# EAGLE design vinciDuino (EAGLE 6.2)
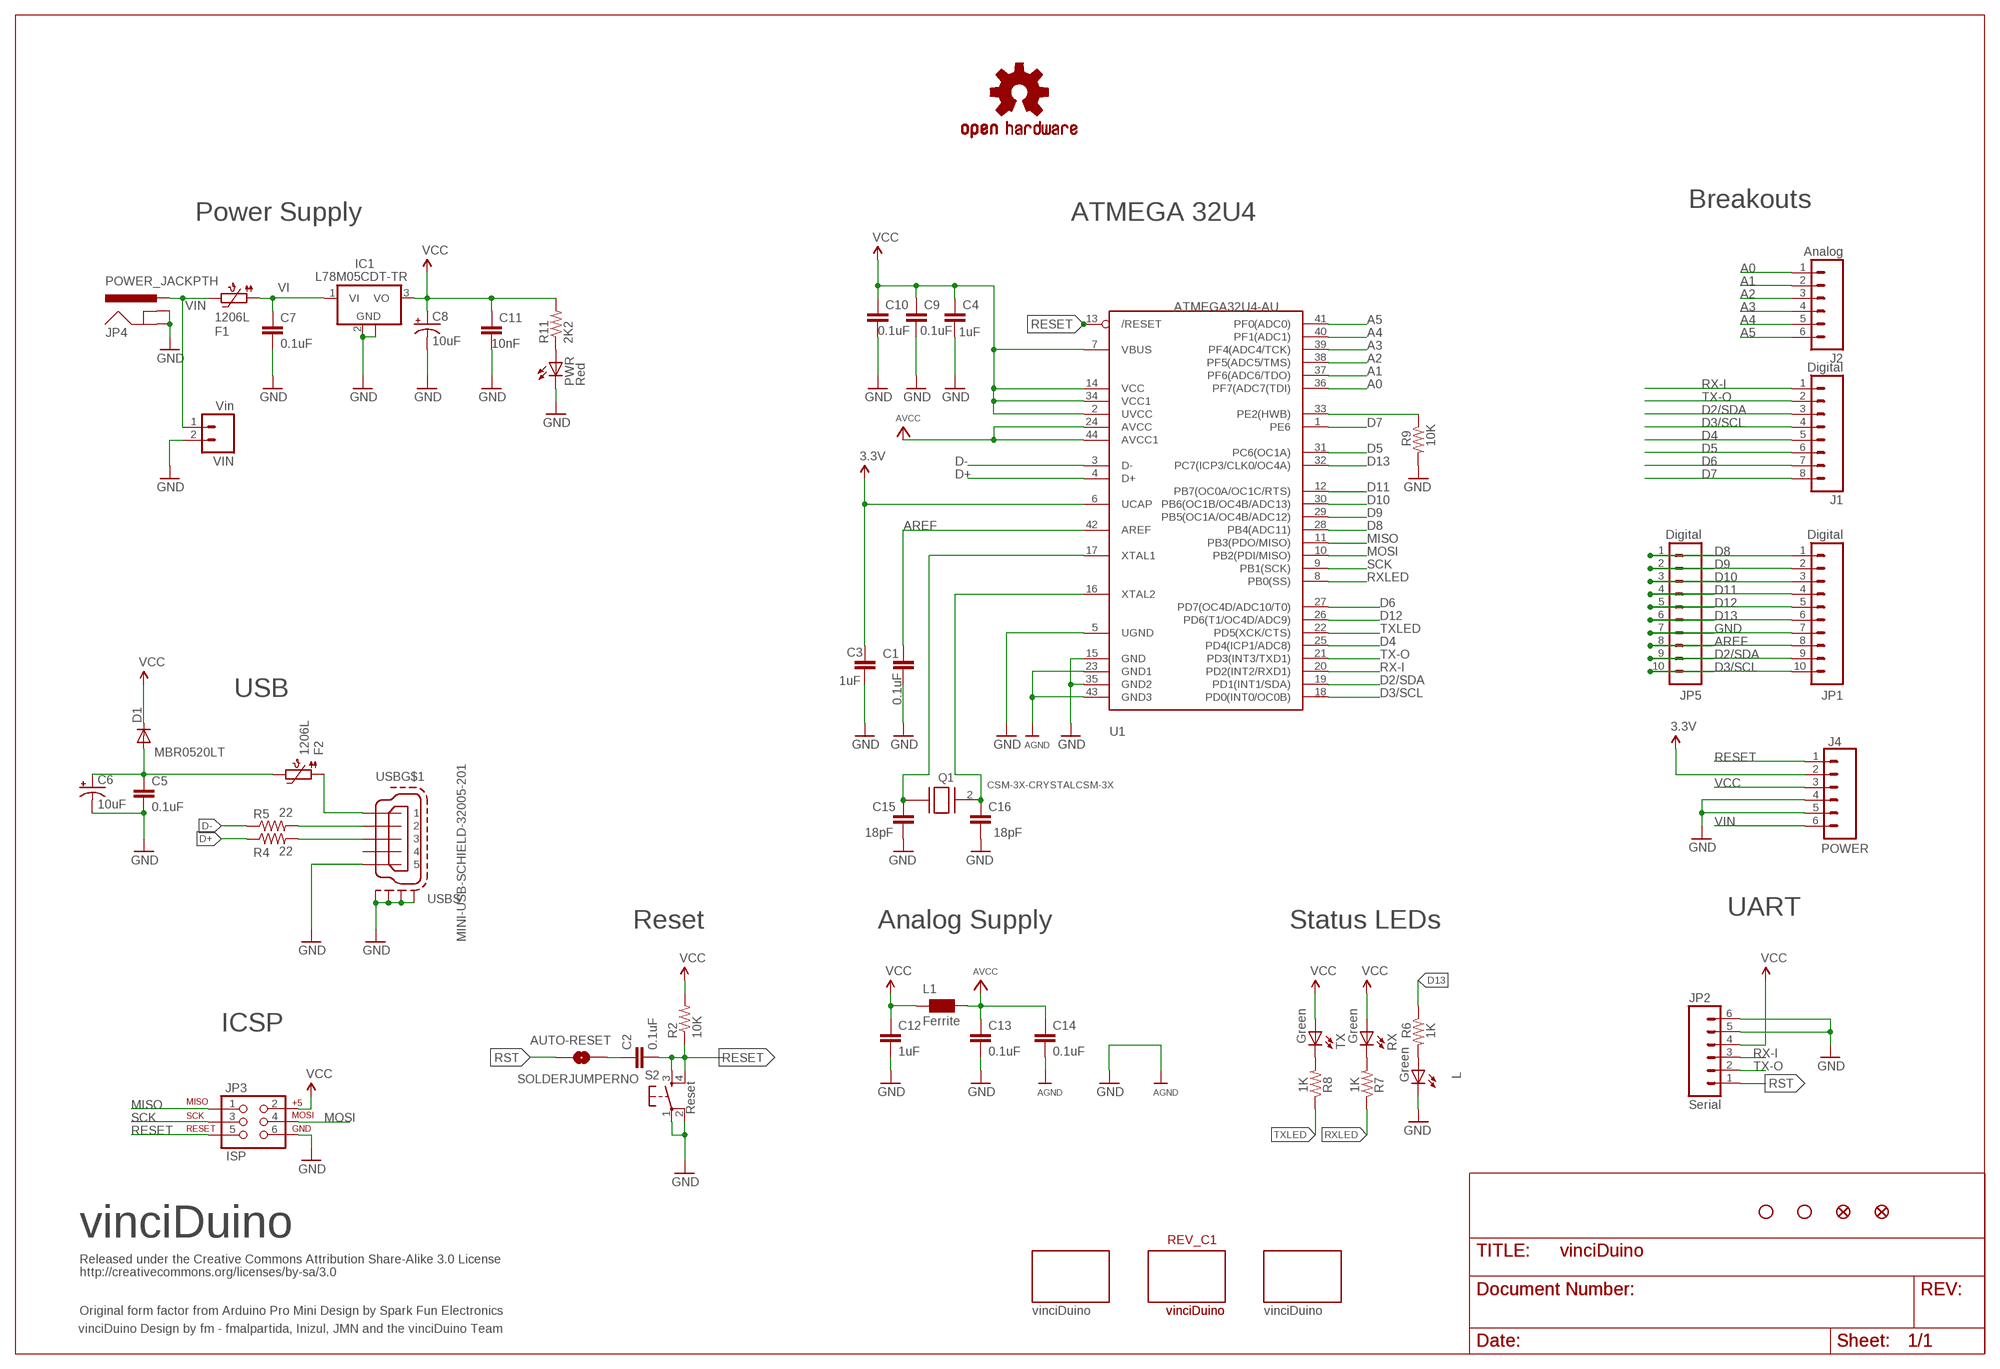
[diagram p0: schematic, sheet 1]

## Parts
AUTO-RESET  SOLDERJUMPERNO  [SJ_2S-NO]
C1  0.1uF  CAP1206  [1206]
C2  0.1uF  CAP1206  [1206]
C3  1uF  CAP1206  [1206]
C4  1uF  CAP1206  [1206]
C5  0.1uF  CAP1206  [1206]
C6  10uF  CAP_POL1206  [EIA3216]
C7  0.1uF  CAP1206  [1206]
C8  10uF  CAP_POL1206  [EIA3216]
C9  0.1uF  CAP1206  [1206]
C10  0.1uF  CAP1206  [1206]
C11  10nF  CAP1206  [1206]
C12  1uF  CAP1206  [1206]
C13  0.1uF  CAP1206  [1206]
C14  0.1uF  CAP1206  [1206]
C15  18pF  CAP1206  [1206]
C16  18pF  CAP1206  [1206]
D1  MBR0520LT  [SOD123]
F1  1206L  PTC1206_L  [1206_PTC]
F2  1206L  PTC1206_L  [1206_PTC]
IC1  L78M05CDT-TR  78XX  [SOT-223-DPAK]
J1  Digital  M081X08  [1X08]
J2  Analog  M06SIP  [1X06]
J4  POWER  M06SIP  [1X06]
JP1  Digital  M10"  [1X10]
JP2  Serial  M06SIP  [1X06]
JP3  ISP  AVR_SPI_PRG_6PTH  [2X3]
JP4  POWER_JACKPTH  [POWER_JACK_PTH]
JP5  Digital  M10"  [1X10]
L  Green  LED1206  [LED-1206]
L1  Ferrite  WE-CBF_1206W  [1206W]
PWR  Red  LED1206  [LED-1206]
Q1  CSM-3X-CRYSTALCSM-3X  [CSM-3X]
R2  10K  R-US_R1206  [R1206]
R4  22  R-US_R1206  [R1206]
R5  22  R-US_R1206  [R1206]
R6  1K  R-US_R1206  [R1206]
R7  1K  R-US_R1206  [R1206]
R8  1K  R-US_R1206  [R1206]
R9  10K  R-US_R1206  [R1206]
R11  2K2  R-US_R1206  [R1206]
REV_C1  vinciDuino  BOARD_INFO_  [ARDUINO_FORUM]
RX  Green  LED1206  [LED-1206]
S2  Reset  TAC_SWITCHSMD  [TACTILE_SWITCH_SMD]
TX  Green  LED1206  [LED-1206]
U1  ATMEGA32U4-AU  [TQFP44]
U$1  VINCIDUINO_  VINCIDUINO_25  [VINCIDUINO]
U$2  FIDUCIAL1X2  [FIDUCIAL-1X2]
U$3  VINCIDUINO_15  [VINCIDUINO_VSMAL]
U$4  FIDUCIAL1X2  [FIDUCIAL-1X2]
U$9  STAND-OFF  [STAND-OFF]
U$10  STAND-OFF  [STAND-OFF]
U$14  OSHW-LOGOS  [OSHW-LOGO-S]
USB  MINI-USB-SCHIELD-32005-201  [32005-201]
VIN  Vin  M021X02_NO_SILK  [1X02_NO_SILK]

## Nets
3.3V: C3.1 J4.2 U1.6(UCAP)
A0: J2.1 U1.36(PF7(ADC7(TDI))
A1: J2.2 U1.37(PF6(ADC6/TDO))
A2: J2.3 U1.38(PF5(ADC5/TMS))
A3: J2.4 U1.39(PF4(ADC4/TCK))
A4: J2.5 U1.40(PF1(ADC1))
A5: J2.6 U1.41(PF0(ADC0))
AREF: C1.2 JP1.8 JP5.8 U1.42(AREF)
AVCC: C13.1 C14.1 L1.2 U1.24(AVCC) U1.44(AVCC1)
D2/SDA: J1.3 JP1.9 JP5.9 U1.19(PD1(INT1/SDA))
D3/SCL: J1.4 JP1.10 JP5.10 U1.18(PD0(INT0/OC0B))
D4: J1.5 U1.25(PD4(ICP1/ADC8))
D5: J1.6 U1.31(PC6(OC1A))
D6: J1.7 U1.27(PD7(OC4D/ADC10/T0))
D7: J1.8 U1.1(PE6)
D8: JP1.1 JP5.1 U1.28(PB4(ADC11))
D9: JP1.2 JP5.2 U1.29(PB5(OC1A/OC4B/ADC12))
D10: JP1.3 JP5.3 U1.30(PB6(OC1B/OC4B/ADC13))
D11: JP1.4 JP5.4 U1.12(PB7(OC0A/OC1C/RTS))
D12: JP1.5 JP5.5 U1.26(PD6(T1/OC4D/ADC9))
D13: JP1.6 JP5.6 R6.1 U1.32(PC7(ICP3/CLK0/OC4A))
D+: R4.1 U1.4(D+)
D-: R5.1 U1.3(D-)
GND: C1.1 C3.2 C4.2 C5.2 C6.C(-) C7.2 C8.C(-) C9.2 C10.2 C11.2 C12.2 C13.2 C14.2 C15.2 C16.2 IC1.2(GND) IC1.4(GND) J4.4 J4.5 JP1.7 JP2.5 JP2.6 JP3.6 JP4.GND JP4.GNDBREAK JP5.7 L.C PWR.C R9.2 S2.1 S2.2 U1.5(UGND) U1.15(GND) U1.23(GND1) U1.35(GND2) U1.43(GND3) USB.5 USB.M1(S:S1) USB.M2(S:S2) USB.M3(S:S3) USB.M4(S:S4) VIN.2 ; supply symbol labelled AGND
MISO: JP3.1 U1.11(PB3(PDO/MISO))
MOSI: JP3.4 U1.10(PB2(PDI/MISO))
N$1: R8.2 TX.C
N$2: R5.2 USB.2
N$3: C16.1 Q1.2 U1.16(XTAL2)
N$4: C15.1 Q1.1 U1.17(XTAL1)
N$5: R4.2 USB.3
N$6: R9.1 U1.33(PE2(HWB))
N$7: L.A R6.2
N$8: AUTO-RESET.2 C2.1
N$9: R7.2 RX.C
N$13: F2.1 USB.1
N$38: PWR.A R11.1
RESET: C2.2 J4.1 JP3.5 R2.1 S2.3 S2.4 U1.13(/RESET)
RST: AUTO-RESET.1 JP2.1
RX-I: J1.1 JP2.3 U1.20(PD2(INT2/RXD1))
RXLED: R7.1 U1.8(PB0(SS))
SCK: JP3.3 U1.9(PB1(SCK))
TX-O: J1.2 JP2.2 U1.21(PD3(INT3/TXD1))
TXLED: R8.1 U1.22(PD5(XCK/CTS))
VBUS: C5.1 C6.A(+) D1.A F2.2
VCC: C4.1 C8.A(+) C9.1 C10.1 C11.1 C12.1 D1.C IC1.3(VO) J4.3 JP2.4 JP3.2 L1.1 R2.2 R11.2 RX.A TX.A U1.2(UVCC) U1.7(VBUS) U1.14(VCC) U1.34(VCC1)
VI [vcc]: C7.1 F1.1 IC1.1(VI)
VIN [vcc]: F1.2 J4.6 JP4.PWR VIN.1
Unconnected: USB.4

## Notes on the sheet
- Breakouts
- Power Supply | ATMEGA 32U4
- USB
- UART
- Reset | Analog Supply | Status LEDs
- ICSP
- vinciDuino
- Released under the Creative Commons Attribution Share-Alike 3.0 License
- http://creativecommons.org/licenses/by-sa/3.0
- Original form factor from Arduino Pro Mini Design by Spark Fun Electronics
- vinciDuino Design by fm - fmalpartida, Inizul, JMN and the vinciDuino Team

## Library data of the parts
AUTO-RESET = SparkFun:SOLDERJUMPER: Solder Jumper
C1-C5 C7 C9-C16 = sparkfun_2:CAP: Capacitor
C6 C8 = SparkFun:CAP_POL: Capacitor Polarized
D1 = diode:MBR0520LT: SCHOTTKY BARRIER RECTIFIER
F1 F2 = microbuilder:PTC: PTC (Resettable Fuse)
IC1 = fmc:78XX
J1 = SparkFun:M08: Header 8 Standard 8-pin 0.1" header. Use with straight break away headers (SKU : PRT-00116), right angle break away headers (PRT-00553), swiss pins (PRT-00743), machine pins (PRT-00117), and female headers (PRT-00115).
J2 J4 JP2 = SparkFun:M06: Header 6 Standard 6-pin 0.1" header. Use with straight break away headers (SKU : PRT-00116), right angle break away headers (PRT-00553), swiss pins (PRT-00743), machine pins (PRT-00117), and female headers (PRT-00115). Molex polarized connector foot print use with SKU : PRT-08094 with associated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
JP1 JP5 = SparkFun:M10: Header 10 Standard 10-pin 0.1" header. Use with straight break away headers (SKU : PRT-00116), right angle break away headers (PRT-00553), swiss pins (PRT-00743), machine pins (PRT-00117), and female headers (PRT-00115).
JP3 = SparkFun:AVR_SPI_PRG_6: AVR ISP 6 Pin This is the reduced ISP connector for AVR programming. Common on Arduino. This footprint will take up less PCB space and can be used with a 10-pin to 6-pin adapter such as SKU: BOB-08508
JP4 = SparkFun:POWER_JACK: Power Jack This is the standard 5.5mm barrel jack for power. The PTH is the most common, proven, reliable, footprint. All others are experimental. The Slot footprint only works if the mill layer is transmitted to the PCB fab house so be warned. Spark Fun Electronics SKU : PRT-00119. Mating wall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
L PWR RX TX = SparkFun:LED: LEDs
L1 = wuerth-elektronik:WE-CBF: SMD EMI Suppression Ferrite Beads
Q1 = fmc:CSM-3X-CRYSTAL
R2 R4-R9 R11 = adafruit:R-US_: RESISTOR, American symbol
REV_C1 = fmc:BOARD_INFO_
S2 = SparkFun:TAC_SWITCH: Momentary Switch Button commonly used for reset or general input. Spark Fun Electronics SKU : COM-00097
U1 = adafruit:ATMEGA32U4: http://www.ladyada.net/library/eagle
U$1 U$3 = fmc:VINCIDUINO_
U$2 U$4 = SparkFun:FIDUCIAL: Fiducial Alignment Points
U$9 U$10 = SparkFun:STAND-OFF: Stand Off
U$14 = SparkFun:OSHW-LOGO: Open Source Hardware Logo This logo indicates the piece of hardware it is found on incorporates a OSHW license and/or adheres to the definition of open source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
USB = con-cypressindustries:MINI-USB-SCHIELD-: MINI USB-B Conector Source: www.cypressindustries.com; OC_FARNELL: unknown; OC_NEWARK: unknown
VIN = SparkFun:M02: Header 2

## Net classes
1 vcc: width 0.254 mm

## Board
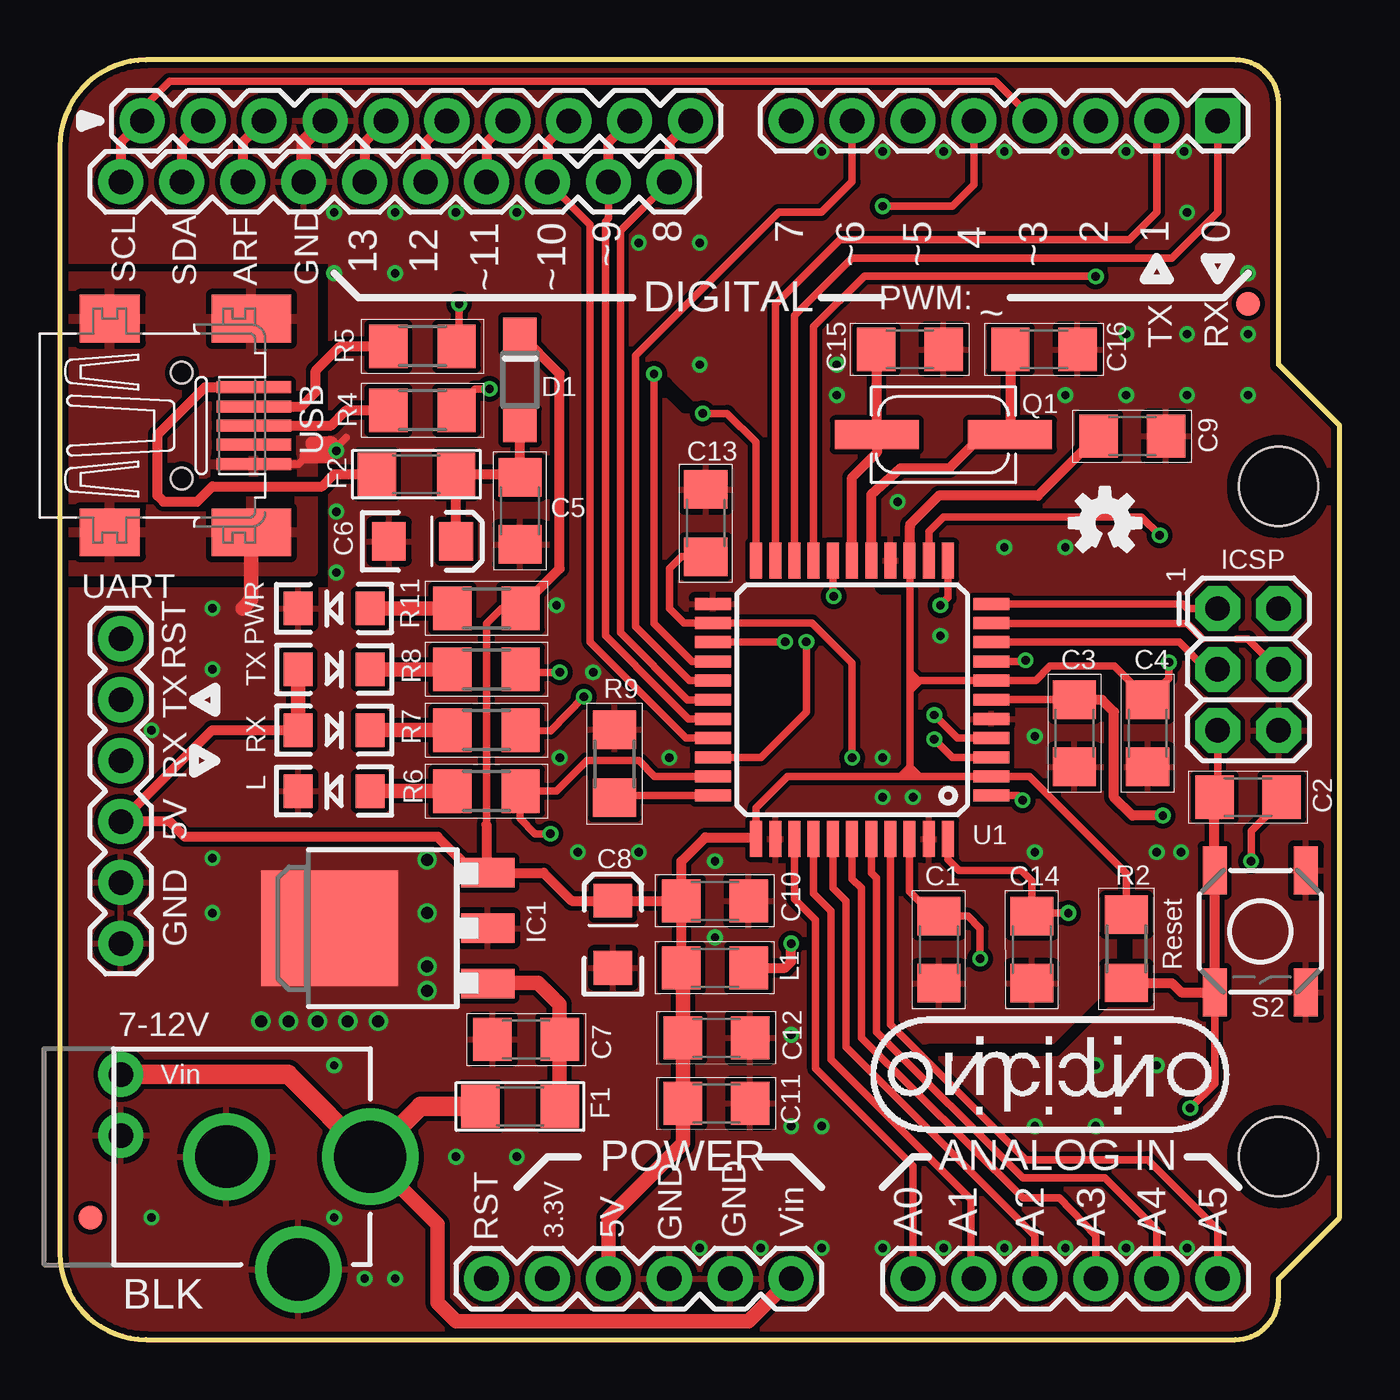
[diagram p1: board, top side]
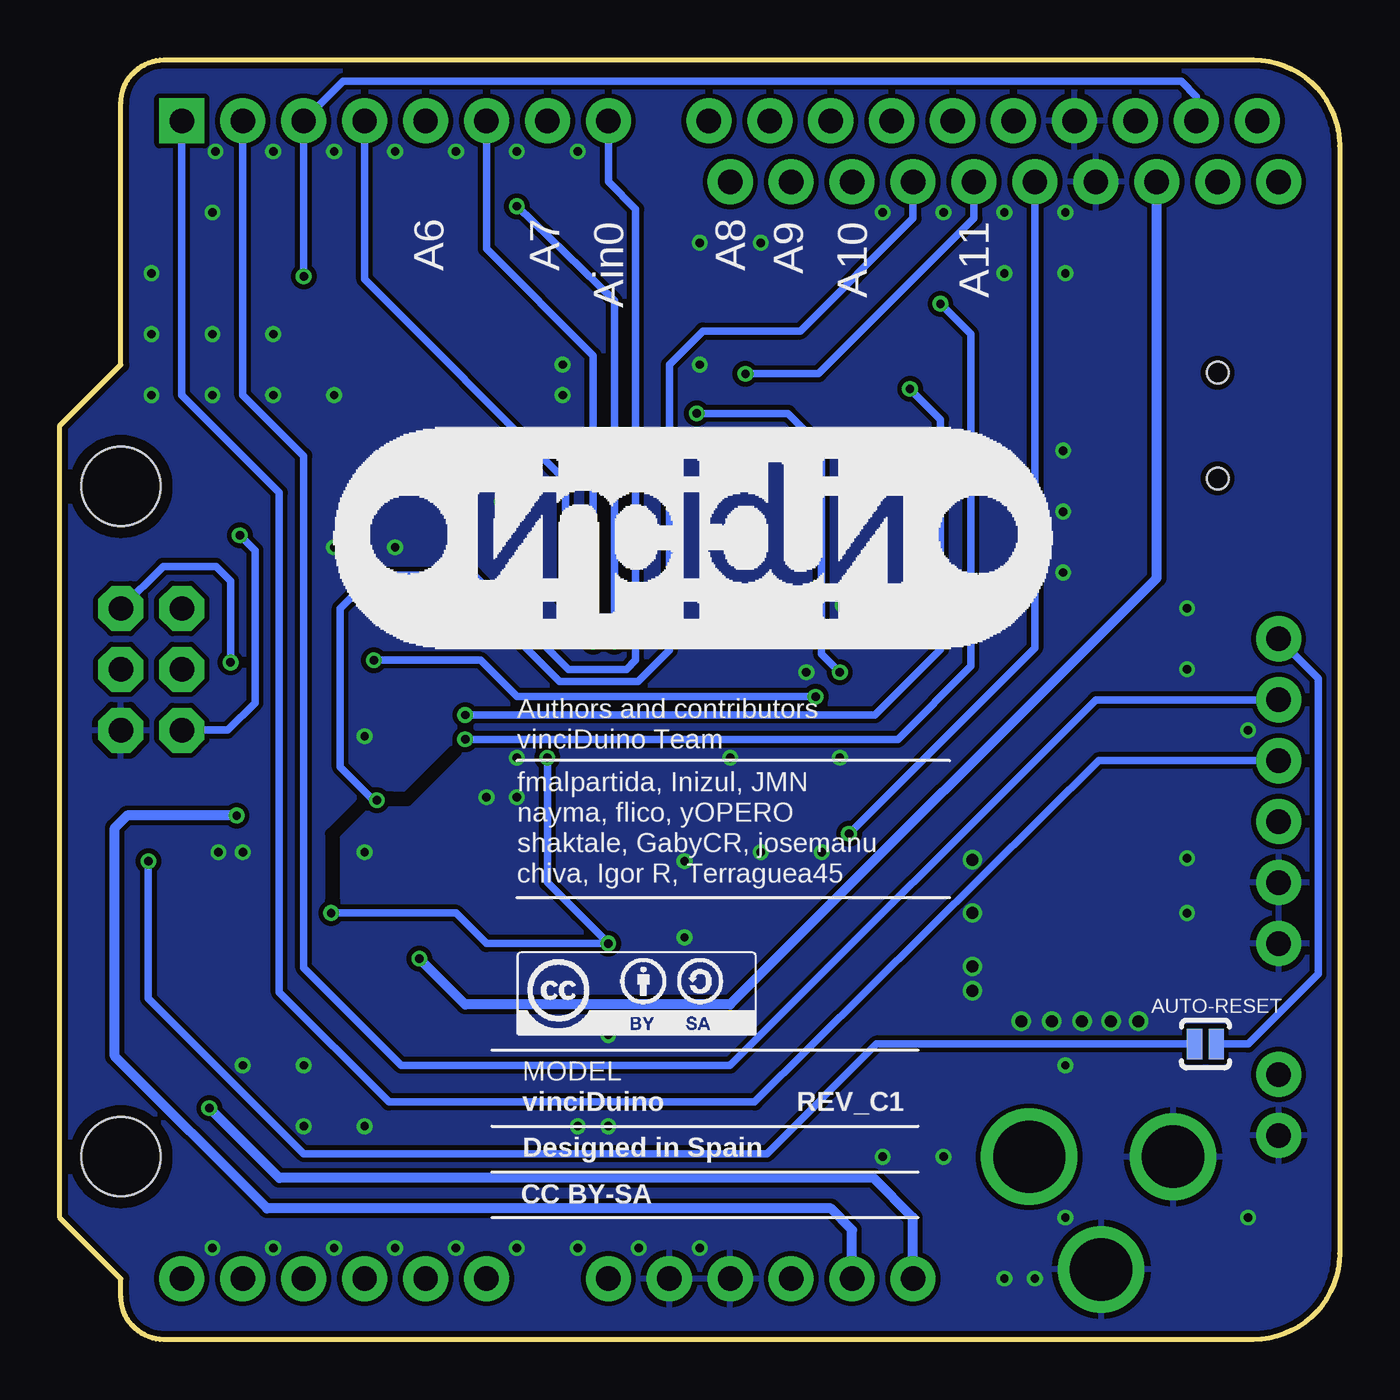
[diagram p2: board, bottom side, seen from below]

Size 53.34 x 53.34 mm. Coordinates in mm from the lower left corner, seen from the top.
Outline: 50.8,40.64 50.8,51.54 arc90 49,53.34 3.59,53.34 arc90 0,49.75 0,3.59 arc90 3.59,0 49,0 arc90 50.8,1.8 50.8,2.54 53.34,5.08 53.34,38.1 50.8,40.64
Copper layers (1*16): Top 0.0356mm / dielectric 1.5011mm / Bottom 0.0356mm
Design rules: minimum track width 6mil, minimum drill 0.35mm, track to track 8mil, track to pad 8mil, pad to pad 8mil, via to via 8mil, smd to smd 8mil, copper to edge 10mil, drill to drill 6mil, minimum pad ring 12mil, minimum via ring 6mil, stop-mask expansion 4mil, vias tented up to drill 25mil, thermal gap 10mil
tRestrict: area 34.3,31.4 to 34.9,31.5; area 25.1,38.9 to 26.2,39.9; area 36.2,12.1 to 43.4,14; area 44.3,15.9 to 44.5,16.8
bRestrict: area 36.8,22.5 to 39.5,24.5; area 40.6,18.3 to 42,22.4

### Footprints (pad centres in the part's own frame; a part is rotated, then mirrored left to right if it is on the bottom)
SJ_2S-NO = smd 0.635 x 1.27: 1 -0.45,0; 2 0.45,0
1206 = smd 1.6 x 1.8: 1 -1.4,0; 2 1.4,0
EIA3216 = smd 1.4 x 1.6: A 1.4,0; C -1.4,0
SOD123 = smd 1.4 x 1.4: A 1.9,0; C -1.9,0
1206_PTC = smd 1.6 x 1.8: 1 -1.654,0; 2 1.654,0
SOT-223-DPAK = smd 1.219 x 2.235: 1 -2.311,-3.099; 2 0,-3.099; 3 2.311,-3.099 | smd 4.826 x 5.715: 4 0,3.493
1X08@1 = drill 1.016 pad 1.88 square: 1 0,0 | drill 1.016 pad 1.88: 2 2.54,0; 3 5.08,0; 4 7.62,0; 5 10.16,0; 6 12.7,0; 7 15.24,0; 8 17.78,0
1X06@1 = drill 1.016 pad 1.88: 1 -6.35,0; 2 -3.81,0; 3 -1.27,0; 4 1.27,0; 5 3.81,0; 6 6.35,0
1X10 = drill 1.016 pad 1.88: 1 0,0; 2 2.54,0; 3 5.08,0; 4 7.62,0; 5 10.16,0; 6 12.7,0; 7 15.24,0; 8 17.78,0; 9 20.32,0; 10 22.86,0
2X3@1 = drill 1.016 pad 1.88 octagon: 1 0,0; 2 0,2.54; 3 2.54,0; 4 2.54,2.54; 5 5.08,0; 6 5.08,2.54
POWER_JACK_PTH@1 = drill 2.6: GND 0,7.7; GNDBREAK 4.7,10.7 | drill 3: PWR 0,13.7
LED-1206 = smd 1.2 x 1.4: A -1.5,0; C 1.5,0
1206W = smd 1.6 x 1.8: 1 -1.4,0; 2 1.4,0
CSM-3X = smd 3.5 x 1.2: 1 2.775,0; 2 -2.775,0
R1206 = smd 1.6 x 1.803: 1 -1.422,0; 2 1.422,0
TACTILE_SWITCH_SMD@1 = smd 2 x 1: 1 -2.54,1.905; 2 2.54,1.905; 3 -2.54,-1.905; 4 2.54,-1.905
TQFP44 = smd 1.5 x 0.5: 1 -5.8,4; 2 -5.8,3.2; 3 -5.8,2.4; 4 -5.8,1.6; 5 -5.8,0.8; 6 -5.8,0; 7 -5.8,-0.8; 8 -5.8,-1.6; 9 -5.8,-2.4; 10 -5.8,-3.2; 11 -5.8,-4; 23 5.8,-4; 24 5.8,-3.2; 25 5.8,-2.4; 26 5.8,-1.6; 27 5.8,-0.8; 28 5.8,0; 29 5.8,0.8; 30 5.8,1.6; 31 5.8,2.4; 32 5.8,3.2; 33 5.8,4 | smd 0.5 x 1.5: 12 -4,-5.8; 13 -3.2,-5.8; 14 -2.4,-5.8; 15 -1.6,-5.8; 16 -0.8,-5.8; 17 0,-5.8; 18 0.8,-5.8; 19 1.6,-5.8; 20 2.4,-5.8; 21 3.2,-5.8; 22 4,-5.8; 34 4,5.8; 35 3.2,5.8; 36 2.4,5.8; 37 1.6,5.8; 38 0.8,5.8; 39 0,5.8; 40 -0.8,5.8; 41 -1.6,5.8; 42 -2.4,5.8; 43 -3.2,5.8; 44 -4,5.8
FIDUCIAL-1X2 = smd 1 x 1: 1 0,0
STAND-OFF@1 = hole 3.302: 0,0
32005-201 = smd 3.1 x 0.5: 1 3,1.6; 2 3,0.8; 3 3,0; 4 3,-0.8; 5 3,-1.6 | smd 2.5 x 2: M1 -3,-4.45; M2 -3,4.45 | smd 3.3 x 2: M3 2.9,4.45; M4 2.9,-4.45 | hole 0.9: 0,2.2; 0,-2.2
1X02_NO_SILK = drill 1.016 pad 1.88: 1 0,0; 2 2.54,0

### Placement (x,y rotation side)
AUTO-RESET  5.59,12.32 180 bottom
C1  36.64,16.26 90 top
C2  49.53,22.61 180 top
C3  42.29,25.27 270 top
C4  45.34,25.27 270 top
C5  19.18,34.54 270 top
C6  15.11,33.27 0 top
C7  19.43,12.51 180 top
C8  23.05,16.89 90 top
C9  44.7,37.66 0 top
C10  27.3,18.29 0 top
C11  27.37,9.84 0 top
C12  27.37,12.57 0 top
C13  26.92,34.04 90 top
C14  40.51,16.26 270 top
C15  35.43,41.27 0 top
C16  41.02,41.27 0 top
D1  19.18,40.01 270 top
F1  19.18,9.72 180 top
F2  14.86,36.07 0 top
IC1  14.73,17.14 90 top
J1  Digital  [1X08@1]  48.26,50.8 180 top
J2  Analog  [1X06@1]  41.91,2.54 0 top
J4  POWER  [1X06@1]  24.13,2.54 0 top
JP1  26.29,50.8 180 top
JP2  Serial  [1X06@1]  2.54,22.86 270 top
JP3  ISP  [2X3@1]  48.26,30.47 270 top
JP4  POWER_JACKPTH  [POWER_JACK_PTH@1]  -0.76,7.62 270 top
JP5  25.4,48.26 180 top
L  11.43,22.86 180 top
L1  27.3,15.49 0 top
PWR  11.43,30.48 180 top
Q1  36.83,37.72 180 top
R2  44.45,16.29 90 top
R4  15.11,38.73 180 top
R5  15.11,41.4 180 top
R6  17.78,22.86 180 top
R7  17.78,25.4 180 top
R8  17.78,27.94 180 top
R9  23.11,24 90 top
R11  17.78,30.48 0 top
REV_C1  26.67,8.89 0 bottom
RX  11.43,25.4 0 top
S2  Reset  [TACTILE_SWITCH_SMD@1]  50.04,17.02 270 top
TX  11.43,27.94 0 top
U1  33.02,26.67 180 top
U$1  41.91,28.83 0 bottom
U$2  1.27,5.08 0 top
U$3  33.78,8.64 0 top
U$4  49.53,43.18 0 top
U$9  STAND-OFF  [STAND-OFF@1]  50.8,35.56 0 top
U$10  STAND-OFF  [STAND-OFF@1]  50.8,7.62 0 top
U$13  [SA-BY]  34.29,12.7 0 bottom
U$14  43.56,34.04 0 top
USB  5.08,38.1 0 top
VIN  2.54,11.05 270 top

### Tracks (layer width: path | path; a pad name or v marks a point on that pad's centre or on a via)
3.3V  (via drill 0.35)
  Top 0.305: C3.1 U1.6
  Top 0.406: v45.97,21.84 44.7,21.84 43.94,22.61 43.94,26.16 43.43,26.67 C3.1
  Bottom 0.406: J4.2 20.32,4.57 21.21,5.46 44.7,5.46 51.05,11.81 51.05,21.34 50.55,21.84 v45.97,21.84
A0
  Top 0.305: U1.36 30.62,18.37 31.5,17.49 31.5,11.3 35.56,7.24 J2.1
A1
  Top 0.305: U1.37 31.42,18.59 32.13,17.88 32.13,11.68 37.97,5.84 37.97,2.67 J2.2
A2
  Top 0.305: U1.38 32.22,18.83 32.77,18.29 32.77,12.19 40.64,4.32 J2.3
A3
  Top 0.305: U1.39 33.02,19.21 33.4,18.83 33.4,12.57 40.13,5.91 41.66,5.91 43.18,4.32 J2.4
A4
  Top 0.305: 33.78,20.83 U1.40 33.82,19.46 34.04,19.24 34.04,12.83 40.13,6.73 43.56,6.73 45.72,4.57 J2.5
A5
  Top 0.305: U1.41 34.62,13.13 40.26,7.49 45.34,7.49 48.26,4.57 J2.6
AREF  (via drill 0.35)
  Top 0.305: U1.42 35.42,18.68 36.58,17.53 36.64,17.53 C1.2 37.85,17.65 38.35,17.14 v38.35,15.88
  Top 0.406: JP1.8 7.62,49.91 JP5.8
  Bottom 0.406: v38.35,15.88 36.45,13.97 25.4,13.97 7.62,31.75 JP5.8
AVCC  (via drill 0.35)
  Top 0.305: U1.44 37.02,20 37.47,19.56 40.07,19.56 40.51,19.11 C14.1 40.51,17.78 v42.04,17.78 | C13.1 25.91,32.64 25.4,32.13 25.4,30.48 26.01,29.87 U1.24 31.34,29.87 33.02,28.19 v33.02,24.26
  Top 0.406: v30.48,16.51 30.48,15.75 30.23,15.49 L1.2
  Bottom 0.305: v30.48,16.51 33.02,19.05 v33.02,24.26 | v30.48,16.51 31.75,17.78 | v42.04,17.78 36.83,17.78 35.56,16.51 v30.48,16.51
D2/SDA  (via drill 0.35)
  Top 0.305: U1.19 31.42,42.22 33.53,44.32 v43.18,44.32
  Top 0.406: JP1.9 5.08,49.91 JP5.9
  Bottom 0.305: JP1.9 5.97,51.82 6.6,52.45 41.53,52.45 J1.3 v43.18,44.32
D3/SCL  (via drill 0.35)
  Top 0.305: JP1.10 3.43,51.31 4.57,52.45 38.99,52.45 J1.4 | U1.18 32.22,31.03 v32.26,30.99
  Top 0.406: JP1.10 2.54,49.91 JP5.10
  Bottom 0.305: v32.26,30.99 32.26,35.81 40.64,44.2 J1.4
D4  (via drill 0.35)
  Top 0.305: U1.25 29.6,29.07 v30.23,29.08 | v34.29,47.24 37.21,47.24 38.1,48.13 J1.5
  Bottom 0.305: v30.23,29.08 30.23,43.31 v34.29,47.24
D5  (via drill 0.35)
  Top 0.305: U1.31 29.22,24.27 31.11,26.16 v31.11,29.08
  Bottom 0.305: v31.11,29.08 31.11,41.02 35.56,45.47 J1.6
D6
  Top 0.305: 26.5,27.47 U1.27 26.25,27.47 24,29.72 24,41.02 29.97,46.99 31.75,46.99 33.02,48.26 J1.7
D7  (via drill 0.35)
  Top 0.305: U1.1 39.94,22.67 v40.13,22.48
  Bottom 0.305: v40.13,22.48 40.26,22.48 41.66,23.88 41.66,30.48 40.26,31.88 36.07,31.88 32.13,27.94 29.72,27.94 29.34,28.32 29.34,47.12 30.48,48.26 J1.8
D8
  Top 0.305: U1.28 26.16,26.67 23.37,29.46 23.37,46.23 JP5.1
  Top 0.406: JP1.1 25.4,49.91 JP5.1
D9
  Top 0.305: 25.27,26.8 22.73,29.34 22.73,46.61 22.86,46.74 JP5.2 | 25.27,26.8 | 25.27,26.8 26.19,25.88 U1.29
  Top 0.406: JP5.2 22.86,49.91 JP1.2
D10
  Top 0.305: U1.30 27.21,25.08 26.1,25.08 22.1,29.08 22.1,46.48 JP5.3
  Top 0.406: JP1.3 20.32,49.91 JP5.3
D11  (via drill 0.35)
  Top 0.305: U1.12 37.02,30.92 v36.7,30.61
  Top 0.406: JP1.4 17.78,49.91 JP5.4
  Bottom 0.305: v36.7,30.61 35.69,30.61 32.51,27.43 29.24,27.43 27.94,28.73 27.94,40.64 26.54,42.04 22.48,42.04 17.78,46.74 JP5.4
D12  (via drill 0.35)
  Top 0.305: U1.26 26.34,28.27 24.77,29.84 v24.77,40.26
  Top 0.406: JP1.5 15.24,49.91 JP5.5
  Bottom 0.305: v24.77,40.26 21.72,40.26 15.24,46.74 JP5.5
D13  (via drill 0.35)
  Top 0.305: U1.32 24.79,23.47 24.13,24.13 21.97,24.13 20.7,22.86 R6.1 19.18,22.84 19.18,21.72 19.81,21.08 v20.45,21.08
  Top 0.406: JP1.6 12.7,49.91 JP5.6
  Bottom 0.305: v20.45,21.08 12.7,28.83 JP5.6
D+  (via drill 0.35)
  Top 0.305: U1.4 37.41,25.07 v36.45,26.04 | 16.51,38.71 R4.1 17.3,39.62 v17.91,39.62
  Bottom 0.305: v36.45,26.04 19.37,26.04 16.64,28.77 16.64,38.35 v17.91,39.62
D-  (via drill 0.35)
  Top 0.305: U1.3 37.2,24.27 v36.45,25.02 | v16.64,43.18 16.64,41.5 R5.1
  Bottom 0.305: v36.45,25.02 18.41,25.02 15.37,28.07 15.37,41.91 v16.64,43.18
GND  (via drill 0.35, 0.5)
  Top 0.305: USB.5 9.96,36.5 10.29,36.83 | 11.18,36.83 11.94,37.59
  Top 0.61: 10.92,50.67 10.16,49.91 JP5.7 | 10.29,36.83 11.18,36.83 | USB.M4 7.98,30.84 7.62,30.48 | 10.54,37.34 11.3,37.34
  other vias: 22.23,27.81 24.13,20.32 21.59,20.32 24.13,45.72 39.37,49.53 26.67,45.72 11.43,44.45 11.43,46.99 40.64,8.89 43.18,8.89 46.99,39.37 49.53,39.37 34.29,49.53 46.99,46.99 30.48,12.7 39.37,33.02 41.91,33.02 41.91,49.53 49.53,44.45 13.97,46.99 13.97,44.45 11.53,31.97 26.67,3.81 29.21,3.81 3.81,5.08 46.99,41.91 49.53,41.91 6.35,20.07 6.35,17.78 26.67,40.64 10.73,13.27 12,13.27 13.27,13.27 15.3,14.54 15.3,15.56 15.3,17.78 8.38,13.27 9.53,13.27 15.3,20 45.72,20.32 46.74,20.32 40.64,25.15 16.51,7.62 19.05,7.62 11.43,11.43 34.29,24.26 36.7,29.34 43.18,11.43 45.72,11.43 34.29,22.61 35.56,22.61 36.83,3.81 39.37,3.81 41.91,3.81 44.45,3.81 46.99,3.81 27.3,19.94 27.3,16.76 31.75,8.89 30.48,8.89 40.64,20.32 11.43,5.08 12.7,2.54 13.97,2.54 20.7,30.61 6.35,30.48 6.35,27.94 11.53,34.51 44.45,49.53 36.83,49.53 46.86,49.53 31.75,49.53 16.51,46.99 19.05,46.99 31.75,3.81 34.29,3.81 25.4,24.26 20.83,24.26 3.81,25.4 44.45,41.91 44.45,39.37 32.38,39.37 34.92,34.92 32.38,40.64 41.91,39.37 11.53,37.05
  pour Top (isolate 0.203): 0,53.34 53.34,53.34 53.34,0 0,0 0,31.24 11.3,31.24 11.3,44.96 0,44.96
  pour Bottom (isolate 0.203): 0,53.34 53.34,53.34 53.34,0 15.88,0.13 10.79,0.13 0,0
  pour Top (no thermals): 7.62,20.32 15.24,20.32 15.24,13.97 7.62,13.97
  pour Top: 0,44.32 10.54,44.32 10.54,32 0,32
MISO
  Top 0.305: U1.11 46.8,30.67 46.99,30.48 JP3.1
MOSI
  Top 0.203: 47.62,29.21 49.05,29.21
  Top 0.305: U1.10 38.84,29.84 46.99,29.84 47.5,29.34 47.62,29.21 | 49.05,29.21 49.52,29.21 JP3.4
N$1
  Top 0.61: TX.C R8.2
N$2
  Top 0.305: 13.97,41.91 13.72,41.66 13.72,41.4 R5.2
  Top 0.406: USB.2 10.07,38.9 10.67,39.5 10.67,40.39 11.68,41.4 R5.2
N$3
  Top 0.406: C16.1 39.62,37.73 Q1.2 38.48,37.72 37.08,36.32 35.05,36.32 33.82,35.22 U1.16
N$4
  Top 0.406: C15.1 34.03,37.72 34.04,37.72 Q1.1 34.05,36.98 33.02,35.94 U1.17
N$5
  Top 0.406: USB.3 11.3,38.1 11.94,38.73 R4.2
N$6
  Top 0.305: U1.33 23.2,22.67 R9.1
N$7
  Top 0.61: L.A R6.2
N$8  (via drill 0.35)
  Top 0.305: C2.1 50.93,22.48 49.66,21.21 v49.66,19.94
  Bottom 0.305: AUTO-RESET.2 19.3,12.32 23.88,7.75 43.18,7.75 49.66,14.22 v49.66,19.94
N$9
  Top 0.61: RX.C R7.2
N$13
  Top 0.406: USB.1 6.04,39.7 4.06,37.72 4.06,35.18 4.32,34.92 5.71,34.92 6.35,35.56 10.92,35.56 11.43,36.07 F2.1
N$38
  Top 0.61: PWR.A R11.1
RESET  (via drill 0.35)
  Top 0.305: U1.13 36.22,33.68 36.83,34.29 45.09,34.29 v45.85,33.53 | JP3.5 48.26,22.74 C2.2 | S2.3 | 48.13,13.97 48.13,10.67 v47.12,9.65 | S2.4 48.01,14.48
  Top 0.406: S2.4 S2.3 | S2.3 C2.2 | R2.1 46.35,14.87 46.74,14.48 48.01,14.48 48.01,14.22 | 48.01,14.22 48.26,13.97 | 48.01,14.22 48.01,14.1 48.13,13.97
  Bottom 0.305: v45.85,33.53 45.21,32.89 45.21,26.54 46.35,25.4 JP3.5
  Bottom 0.406: J4.1 17.78,5.08 19.43,6.73 44.2,6.73 v47.12,9.65
RST
  Bottom 0.305: JP2.1 0.89,27.56 0.89,15.24 3.81,12.32 AUTO-RESET.1 5.21,12.32
RX-I
  Top 0.305: U1.20 30.62,42.69 33.02,45.09 46.35,45.09 48.26,46.99 J1.1
  Bottom 0.305: JP2.3 10.03,24.13 24.38,9.91 39.62,9.91 44.2,14.48 44.2,35.31 48.26,39.37 J1.1
RXLED  (via drill 0.35)
  Top 0.305: U1.8 40.34,28.27 v40.26,28.32 | v21.84,26.8 20.45,25.38 R7.1
  Bottom 0.305: v40.26,28.32 35.81,28.32 34.29,26.8 v21.84,26.8
SCK
  Top 0.305: U1.9 46.65,29.07 47.78,27.94 JP3.3
TX-O
  Top 0.305: U1.21 29.82,43.16 32.51,45.85 44.58,45.85 45.72,46.99 J1.2
  Bottom 0.305: JP2.2 10.16,26.67 25.4,11.43 39.12,11.43 43.18,15.49 43.18,36.83 45.72,39.37 J1.2
TXLED  (via drill 0.35)
  Top 0.305: R8.1 19.33,27.81 v20.83,27.81 | v26.8,38.61 27.81,38.61 29.02,37.4 U1.22
  Bottom 0.305: v26.8,38.61 22.99,38.61 21.59,37.21 21.59,28.57 v20.83,27.81
VBUS
  Top 0.406: D1.A C5.1 19.05,36.07 F2.2 C6.A
VCC  (via drill 0.35)
  Top 0.254: 35.43,33.91 35.43,33.98
  Top 0.305: 35.56,23.47 30.33,23.47 29.02,22.16 U1.34 28.96,20.93 | 35.56,23.47 U1.2 40.41,23.47 44.45,19.43 R2.2 | 35.43,23.88 35.43,23.6 35.56,23.47 | 35.43,23.88 35.43,27.05 | 35.43,27.05 35.43,27.3 | 35.43,27.3 35.43,27.81 | 35.43,27.81 35.43,32.46 U1.14 35.43,32.48 | 35.43,27.3 35.6,27.47 U1.7 40.68,27.47 41.27,28.07 43.95,28.07 C4.1 46.23,27.56 v46.23,28.23 | 35.43,27.81 35.81,27.43 35.43,27.05 | 35.43,23.88 35.81,23.5 | 35.43,23.88 35.05,23.5 | R11.2 18.41,30.48 17.78,29.84 17.78,21.46
  Top 0.406: R11.2 19.2,30.5 20.83,32.13 20.83,40.25 D1.C | 28.96,20.93 26.9,20.93 25.91,19.94 C10.1 | C10.1 C8.A 21.34,18.29 20.17,19.46 IC1.3 | C10.1 25.91,15.29 L1.1 | 35.43,32.48 35.43,33.91 | RX.A 6.35,25.4 JP2.4 4.57,21.59 5.21,20.95 15.75,20.95 17.4,19.3 17.02,19.3 17.14,19.43 17.09,19.43 IC1.3 | 17.78,19.43 17.07,19.43 IC1.3 | 17.78,21.46 17.78,19.41 IC1.3 | C9.1 42.61,37.02 40.77,35.18 36.64,35.18 35.43,33.98
  Top 0.61: L1.1 25.86,15.34 25.75,15.34 25.53,15.11 | RX.A TX.A | J4.3 22.86,5.08 25.97,8.19 C11.1 C12.1 25.97,14.67 25.53,15.11 | 25.53,15.11 25.4,15.24
  Bottom 0.305: v46.23,28.23 46.23,31.62 46.83,32.23 49.05,32.23 JP3.2
VI
  Top 0.61: IC1.1 17.09,14.86 19.94,14.86 20.83,13.97 C7.1 20.83,10.16 20.95,10.03 20.95,9.97 F1.1
VIN
  Top 0.61: J4.6 28.7,0.76 16.51,0.76 15.75,1.52 15.75,4.81 JP4.PWR
  Top 0.813: F1.2 15.03,9.72 JP4.PWR 9.51,11.05 VIN.1

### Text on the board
tPlace: 8 | 7 | 2 | 1 | 0 | ~9 | ~6 | ~5 | 4 | ~3 | SCL | SDA | ARF | GND | 13 | 12 | ~11 | ~10 | PWM: | DIGITAL | ~ | TX | RX | UART | 1 | ICSP | RST | TX | RX | 5V | GND | Reset | 7-12V | Vin | POWER | ANALOG IN | RST | 3.3V | 5V | GND | GND | Vin | A0 | A1 | A2 | A3 | A4 | A5 | BLK
bPlace: Authors and contributors | vinciDuino Team | fmalpartida, Inizul, JMN | nayma, flico, yOPERO | shaktale, GabyCR, josemanu | chiva, Igor R, Terraguea45
bNames: A11 | A10 | A9 | A8 | Ain0 | A7 | A6
tDocu: Released under the Creative Commons Attribution Share-Alike 3.0 License | http://creativecommons.org/licenses/by-sa/3.0 | vinciDuino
